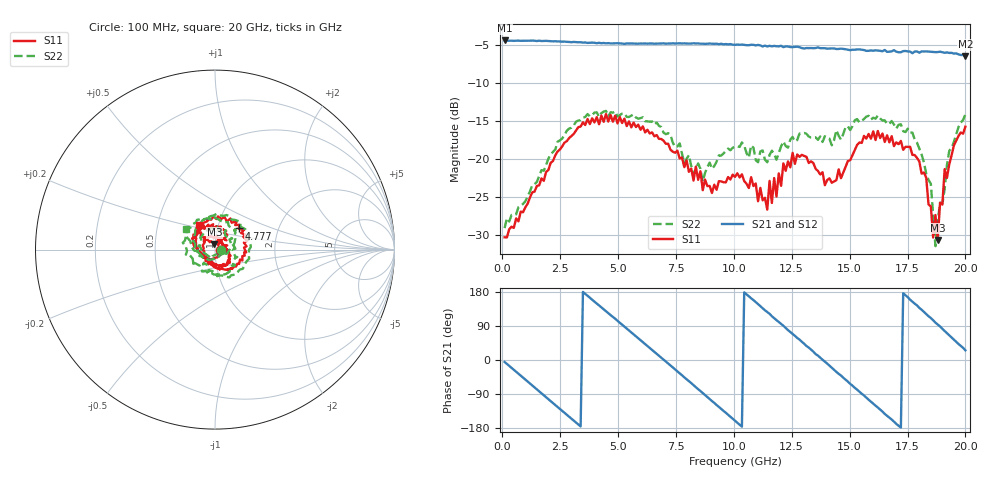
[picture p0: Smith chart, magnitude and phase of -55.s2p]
!Agilent Technologies,N5230C,MY49001569,A.09.33.09
!Agilent N5230C: A.09.33.09
!Date: Tuesday, July 21, 2015 11:36:15
!Correction: S11(Full 2 Port(1,2))
!S21(Full 2 Port(1,2))
!S12(Full 2 Port(1,2))
!S22(Full 2 Port(1,2))
!S2P File: Measurements: S11, S21, S12, S22:
# Hz S  dB  R 50
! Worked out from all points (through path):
!   201 points, 100 MHz to 20 GHz, reference 50 ohm
!   highest |S21| = -4.37 dB at 100 MHz (marker M1); lowest = -6.4 dB at 20 GHz (marker M2)
!   group delay of S21, straight-line fit = 146 ps
!   lowest |S11| = -30.6 dB at 18.81 GHz (marker M3), VSWR 1.06, Z = 49.6 + j2.9 ohm
!   |S11| at or under -10 dB: start of sweep to end of sweep
!   |S22| runs from -31.4 to -13.6 dB; largest |S21 - S12| = 0.016
!   S11 on the Smith chart (normalised r, x): 100 MHz: 1.06, -0.01; 4.777 GHz: 1.26, +0.31; 20 GHz: 0.81, +0.23
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1e8  -30.28 -8.1  -4.37 -5.2  -4.36 -5.0  -29.07 -7.3
1.7915e9  -22.85 -157.0  -4.43 -93.0  -4.44 -92.8  -21.52 -157.0
3.483e9  -15.15 104.5  -4.66 179.7  -4.68 179.3  -14.52 97.6
4.7765e9  -15.06 41.8  -4.75 113.7  -4.76 113.7  -13.87 29.5
5.672e9  -15.18 -5.0  -4.78 67.8  -4.78 67.8  -14.11 -14.8
6.7665e9  -17.32 -48.5  -4.77 11.3  -4.78 11.5  -15.61 -66.8
8.458e9  -22.71 -127.0  -4.76 -77.0  -4.75 -76.7  -20.56 -157.3
1.005e10  -22.32 120.4  -4.94 -160.4  -4.92 -160.2  -18.37 101.5
1.1443e10  -26.63 34.3  -5.16 126.5  -4.91 126.5  -20.40 16.0
1.19405e10  -21.87 -12.0  -5.15 100.3  -5.13 99.8  -19.21 -12.5
1.3433e10  -20.50 -70.5  -5.39 22.1  -5.30 21.6  -17.14 -89.8
1.39305e10  -23.42 -108.4  -5.39 -4.4  -5.42 -4.5  -16.97 -120.6
1.5224e10  -18.77 173.0  -5.58 -73.5  -5.72 -73.6  -14.87 168.7
1.67165e10  -17.77 108.8  -5.84 -152.1  -5.82 -151.8  -15.35 89.5
1.801e10  -20.29 49.1  -5.98 137.6  -5.89 138.7  -18.59 21.2
1.85075e10  -26.22 59.7  -5.86 110.8  -5.91 110.5  -23.22 -19.9
1.8607e10  -30.30 53.0  -5.88 105.0  -5.88 104.5  -27.42 -24.4
1.87065e10  -27.34 82.8  -5.91 98.6  -5.95 99.3  -31.44 -64.1
1.8806e10  -30.64 96.1  -5.90 93.5  -6.01 93.5  -28.11 -110.8
1.91045e10  -21.30 127.8  -5.99 76.5  -6.05 76.0  -23.92 -162.7
1.93035e10  -20.67 130.5  -6.01 64.8  -6.05 64.9  -18.89 -176.3
2e10  -15.72 122.4  -6.43 25.6  -6.40 26.1  -14.11 145.2
